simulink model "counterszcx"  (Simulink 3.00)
settings: Solver=FixedStepDiscrete  SolverMode=MultiTasking  StartTime=0.0  StopTime=2  FixedStep=.01  RelTol=1e-3  AbsTol=1e-6

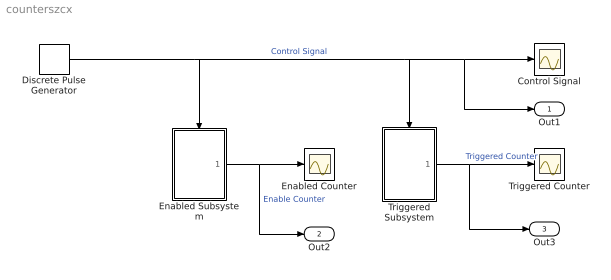
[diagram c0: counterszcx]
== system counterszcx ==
  Control Signal : Scope
  Discrete Pulse Generator : DiscretePulseGenerator  Amplitude=1  Period=4  PulseWidth=2  PhaseDelay=0  SampleTime=0.1
  Enabled Counter : Scope
  Enabled Subsystem : Subsystem
  Triggered Counter : Scope
  Triggered Subsystem : Subsystem
  Out1 : Outport  Port=1
  Out2 : Outport  Port=2
  Out3 : Outport  Port=3
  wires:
  Discrete Pulse Generator/1 -> Enabled Subsystem/Enable, Triggered Subsystem/Trigger, Control Signal/1, Out1/1  "Control Signal"
  Triggered Subsystem/1(tOut) -> Triggered Counter/1, Out3/1  "Triggered Counter"
  Enabled Subsystem/1(eOut) -> Enabled Counter/1, Out2/1  "Enable Counter"

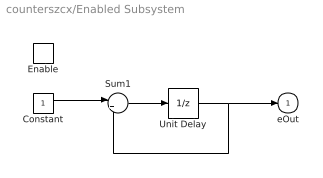
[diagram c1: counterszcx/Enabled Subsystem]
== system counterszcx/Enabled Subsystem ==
  Enable : EnablePort  StatesWhenEnabling=reset
  Constant : Constant  Value=1
  Sum1 : Sum  Inputs=|++  SaturateOnIntegerOverflow=on
  Unit Delay : UnitDelay  X0=0  SampleTime=.01
  eOut : Outport  Port=1  InitialOutput=0
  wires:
  Sum1/1 -> Unit Delay/1
  Constant/1 -> Sum1/1
  Unit Delay/1 -> eOut/1, Sum1/2

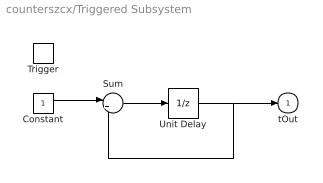
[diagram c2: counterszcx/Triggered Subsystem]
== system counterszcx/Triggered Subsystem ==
  Trigger : TriggerPort  TriggerType=rising  OutputDataType=auto
  Constant : Constant  Value=1
  Sum : Sum  Inputs=|++  SaturateOnIntegerOverflow=on
  Unit Delay : UnitDelay  X0=0  SampleTime=-1
  tOut : Outport  Port=1  OutputWhenDisabled=reset  InitialOutput=0
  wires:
  Sum/1 -> Unit Delay/1
  Constant/1 -> Sum/1
  Unit Delay/1 -> tOut/1, Sum/2
